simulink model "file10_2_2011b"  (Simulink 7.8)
settings: Solver=ode4  StartTime=0.0  StopTime=11  FixedStep=1e-3  RelTol=1e-3

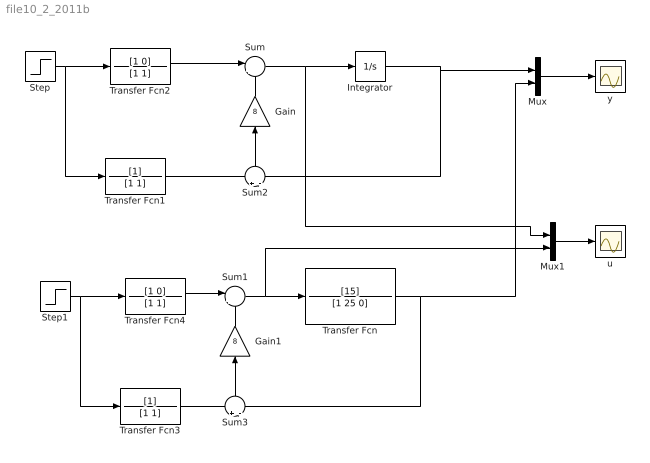
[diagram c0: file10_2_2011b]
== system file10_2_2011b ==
  Gain : Gain  Gain=8
  Gain1 : Gain  Gain=8
  Integrator : Integrator
  Mux : Mux  Inputs=2
  Mux1 : Mux  Inputs=2
  Step : Step  SampleTime=0
  Step1 : Step  SampleTime=0
  Sum : Sum  Inputs=|++
  Sum1 : Sum  Inputs=|++
  Sum2 : Sum  Inputs=+|-
  Sum3 : Sum  Inputs=+|-
  Transfer Fcn : TransferFcn  Numerator=[15]  Denominator=[1 25 0]
  Transfer Fcn1 : TransferFcn  Denominator=[1 1]
  Transfer Fcn2 : TransferFcn  Numerator=[1 0]  Denominator=[1 1]
  Transfer Fcn3 : TransferFcn  Denominator=[1 1]
  Transfer Fcn4 : TransferFcn  Numerator=[1 0]  Denominator=[1 1]
  u : Scope
  y : Scope
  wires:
  Integrator/1 -> Sum2/2, Mux/1
  Step/1 -> Transfer Fcn1/1, Transfer Fcn2/1
  Transfer Fcn1/1 -> Sum2/1
  Gain/1 -> Sum/2
  Sum2/1 -> Gain/1
  Sum/1 -> Integrator/1, Mux1/1
  Transfer Fcn2/1 -> Sum/1
  Transfer Fcn/1 -> Sum3/2, Mux/2
  Step1/1 -> Transfer Fcn3/1, Transfer Fcn4/1
  Transfer Fcn3/1 -> Sum3/1
  Gain1/1 -> Sum1/2
  Sum3/1 -> Gain1/1
  Transfer Fcn4/1 -> Sum1/1
  Sum1/1 -> Transfer Fcn/1, Mux1/2
  Mux/1 -> y/1
  Mux1/1 -> u/1
